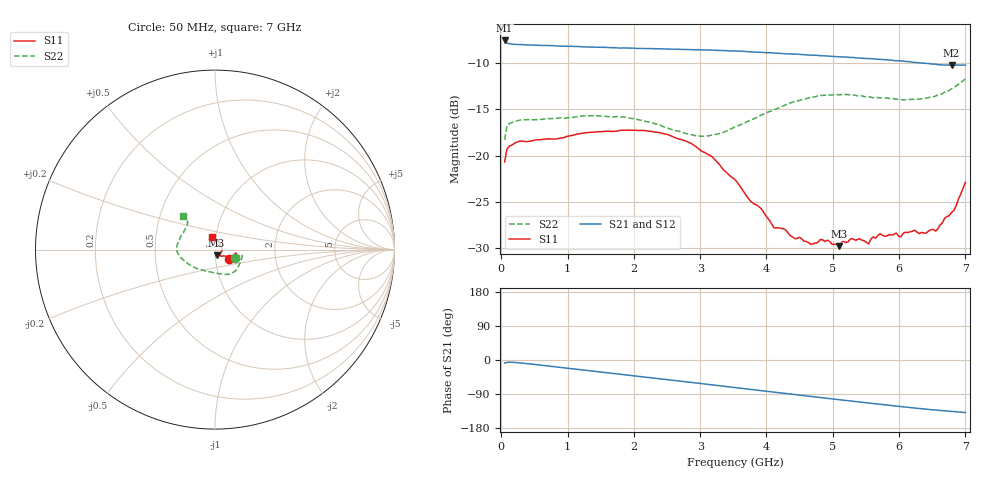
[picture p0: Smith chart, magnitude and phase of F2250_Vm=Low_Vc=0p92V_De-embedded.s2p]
! Integrated Device Technology
! Corporate Headquarters
! 6024 Silver Creek Valley Road
! San Jose, CA 95138  USA
! Phone:  1-408-284-8200
! Toll Free:  1-800-223-1366
! Webpage:  http://www.idt.com/
! Timing and RF Division
! 515 Groton Road, Suite 102
! Westford, MA 01886-6024
! Device:  F2250
! Description: Voltage Variable RF Attenuator
! Frequency:  50.0 -  6000.00 MHz
! Package:  3x3 mm Thin QFN Plastic Package: 16 pin
! Ports:  2 RF, 3 DC
!  Pin  1  = GND
!  Pin  2  = NC
!  Pin  3  = RF1  = Port 1
!  Pin  4  = NC
!  Pin  5  = GND
!  Pin  6  = GND
!  Pin  7  = GND
!  Pin  8  = GND
!  Pin  9  = NC
!  Pin 10  = RF2  = Port 2
!  Pin 11  = NC
!  Pin 12  = GND
!  Pin 13  = GND
!  Pin 14  = VCNTRL
!  Pin 15  = VDD
!  Pin 16  = VMODE
! Vcntrl:  0.920 Volts
! Vmode:  +0.000 Volts
! Vdd:  +3.30  Volts
! Current:  1.179 mA
! Data:  The device was measured on a the F2250 evaluation board which has
!  individual transmission lines to the RF pins.  Data was collected
!  using a calibrated network analyzer.  The evaluation board was
!  de-embedded using a TRL calibration technique.
!  The reference plane is the edge of the package pin.
! Misc:  SN 10
!  Action Tracker AT0258
! Date Measured:  2014-11-26
! Date:  2015-10-15  MJV
! Note:
!  Integrated Device Technology supplies this data as a sample of measured
!  data at the package pin for this product.  Your particular data for this
!  product may vary.
!  Data was taken at 25 degrees C.
!  Integrated Device Technology reserves the right to change this data at anytime.
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# GHz S dB R 50
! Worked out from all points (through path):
!   201 points, 50 MHz to 7 GHz, reference 50 ohm
!   highest |S21| = -7.59 dB at 50 MHz (marker M1); lowest = -10.3 dB at 6.792 GHz (marker M2)
!   group delay of S21, straight-line fit = 55.5 ps
!   lowest |S11| = -29.8 dB at 5.089 GHz (marker M3), VSWR 1.07, Z = 50.8 - j3.19 ohm
!   |S11| at or under -10 dB: start of sweep to end of sweep
!   |S22| runs from -18.3 to -11.7 dB; largest |S21 - S12| = 0.001
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0.05  -20.69 -35.3  -7.59 -8.2  -7.58 -8.2  -18.30 -23.1
0.08475  -19.31 -17.7  -7.86 -6.3  -7.85 -6.2  -16.82 -12.7
0.2585  -18.48 -9.8  -8.02 -7.3  -8.04 -7.3  -16.22 -12.8
1.2315  -17.58 -22.5  -8.28 -26.3  -8.27 -26.3  -15.72 -42.2
1.857  -17.27 -24.5  -8.39 -38.7  -8.40 -38.7  -15.84 -56.6
2.37825  -17.51 -23.6  -8.48 -49.1  -8.47 -49.1  -16.67 -70.1
3.00375  -19.44 -23.6  -8.60 -61.9  -8.61 -61.9  -17.91 -99.4
3.1775  -20.11 -25.3  -8.63 -65.5  -8.64 -65.5  -17.78 -110.4
3.525  -22.59 -31.4  -8.72 -72.8  -8.73 -72.8  -16.92 -130.6
3.942  -25.91 -45.2  -8.88 -81.4  -8.88 -81.4  -15.57 -150.4
4.11575  -27.78 -55.2  -8.95 -84.9  -8.95 -85.0  -15.05 -157.3
4.7065  -29.49 -79.9  -9.18 -97.0  -9.17 -97.0  -13.69 -173.6
4.81075  -29.05 -81.1  -9.22 -99.0  -9.23 -99.0  -13.52 -175.7
5.08875  -29.76 -74.9  -9.35 -104.6  -9.35 -104.6  -13.44 177.8
5.29725  -28.94 -63.8  -9.42 -108.7  -9.43 -108.7  -13.45 173.2
5.5405  -29.51 -51.6  -9.54 -113.5  -9.53 -113.6  -13.64 166.8
5.61  -28.76 -47.4  -9.56 -114.9  -9.56 -114.9  -13.76 165.2
5.85325  -28.50 -31.0  -9.70 -119.6  -9.70 -119.6  -13.84 158.7
6.54825  -28.14 43.4  -10.14 -132.1  -10.15 -132.2  -13.59 137.0
6.7915  -26.13 77.1  -10.26 -135.5  -10.25 -135.6  -12.77 133.6
6.861  -25.40 86.8  -10.25 -136.6  -10.24 -136.7  -12.51 133.7
7  -22.89 104.6  -10.24 -138.8  -10.25 -138.8  -11.73 133.4
